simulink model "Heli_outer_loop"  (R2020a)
settings: Solver=FixedStepDiscrete  StartTime=0.0  StopTime=10.0  FixedStep=0.01  RelTol=1e-3  EnableMultiTasking=on
model workspace (MAT data in the model file):
  Ts = 0.01
undefined symbols (not defined in the file or in its folder): DiscIntNeverNeededParam
libraries: simulink x1

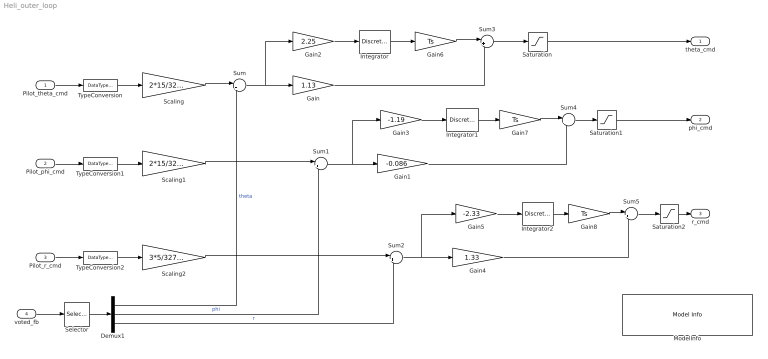
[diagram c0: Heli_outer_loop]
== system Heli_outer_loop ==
  Pilot_theta_cmd : Inport  RequirementInfo={} %GIDa_c6e8f1b9_b611_43b0_b09b_f7299b128b80  OutMin=-32768  OutMax=32767  OutDataTypeStr=int16  PortDimensions=1  SampleTime=0.01
  Pilot_phi_cmd : Inport  RequirementInfo={} %GIDa_de5a2227_6f1d_448c_bc8c_e667ffb26dd8  Port=2  OutMin=-32768  OutMax=32767  OutDataTypeStr=int16  PortDimensions=1  SampleTime=0.01
  Pilot_r_cmd : Inport  RequirementInfo={} %GIDa_bd336e52_072b_4081_8e24_5224b916f056  Port=3  OutMin=-32768  OutMax=32767  OutDataTypeStr=int16  PortDimensions=1  SampleTime=0.01
  voted_fb : Inport  RequirementInfo={} %GIDa_40b9d006_7ccb_49cb_a6ac_aff381845bc4  Port=4  OutMin=-180  OutMax=180  OutDataTypeStr=double  PortDimensions=5  SampleTime=0.01
  Demux1 : Demux  RequirementInfo={} %GIDa_0f7e0ef4_98d4_4326_93b8_613d0164b4b2  Outputs=3
  Gain : Gain  RequirementInfo={} %GIDa_38b33631_7d46_423a_acdb_ff93985993a9  Gain=1.13
  Gain1 : Gain  RequirementInfo={} %GIDa_225d17d5_1a8e_4842_95f8_ce528d38517d  Gain=-0.086
  Gain2 : Gain  RequirementInfo={} %GIDa_ec453ec5_c5c0_44d5_948e_65c93ddaef7c  Gain=2.25
  Gain3 : Gain  RequirementInfo={} %GIDa_943f3cbe_3937_44aa_af38_ec7fec40805c  Gain=-1.19
  Gain4 : Gain  RequirementInfo={} %GIDa_d845b47e_971b_498b_bbe3_d6058df44643  Gain=1.33
  Gain5 : Gain  RequirementInfo={} %GIDa_0a451155_7422_4e41_b41b_ac8de7a0f7bc  Gain=-2.33
  Gain6 : Gain  RequirementInfo={} %GIDa_ec453ec5_c5c0_44d5_948e_65c93ddaef7c  Gain=Ts
  Gain7 : Gain  Gain=Ts
  Gain8 : Gain  Gain=Ts
  Integrator : DiscreteIntegrator  RequirementInfo={} %GIDa_dac8ce2c_b2e5_46af_8a5f_5c149ac95a38  IntegratorMethod=Accumulation: Forward Euler  SampleTime=-1  LimitOutput=on  UpperSaturationLimit=10  LowerSaturationLimit=-10  ICPrevOutput=DiscIntNeverNeededParam  ICPrevScaledInput=DiscIntNeverNeededParam
  Integrator1 : DiscreteIntegrator  RequirementInfo={} %GIDa_c2996118_add0_406e_b8f4_096077f2e691  IntegratorMethod=Accumulation: Forward Euler  SampleTime=-1  LimitOutput=on  UpperSaturationLimit=10  LowerSaturationLimit=-10  ICPrevOutput=DiscIntNeverNeededParam  ICPrevScaledInput=DiscIntNeverNeededParam
  Integrator2 : DiscreteIntegrator  RequirementInfo={} %GIDa_cf0bee46_0c0a_47b2_81ab_c926ffb37de9  IntegratorMethod=Accumulation: Forward Euler  SampleTime=-1  LimitOutput=on  UpperSaturationLimit=10  LowerSaturationLimit=-10  ICPrevOutput=DiscIntNeverNeededParam  ICPrevScaledInput=DiscIntNeverNeededParam
  ModelInfo : simulink/Model-Wide Utilities/Model Info  Frame=on  DisplayStringWithTags=|  HorizontalTextAlignment=Center  LeftAlignmentValue=0.5
      | Model Name: %<ModelName>
      | Model Version: %<ModelVersion>
      | Last Modified: %<LastModificationDate>
      | 
      | Copyright 2016 The MathWorks, Inc.
  Saturation : Saturate  RequirementInfo={} %GIDa_cd349ed3_fa5b_45c3_8aec_effea4668e69  UpperLimit=30  LowerLimit=-30
  Saturation1 : Saturate  RequirementInfo={} %GIDa_cdaf265c_9ec2_4b78_ae7f_0c72f3978ef0  UpperLimit=30  LowerLimit=-30
  Saturation2 : Saturate  RequirementInfo={} %GIDa_b0697b07_104a_4fe5_acf7_d696411481f0  UpperLimit=30  LowerLimit=-30
  Scaling : Gain  Gain=2*15/32767
  Scaling1 : Gain  Gain=2*15/32767
  Scaling2 : Gain  Gain=3*5/32767
  Selector : Selector  RequirementInfo={} %GIDa_e0faeade_0420_4977_bcc4_4057337ee888  InputPortWidth=5  IndexOptions=Index vector (dialog)  Indices=[1 2 3]  OutputSizes=1
  Sum : Sum  RequirementInfo={} %GIDa_aef1367a_fa96_4043_ad47_b91e9938bcbc  Inputs=|+-  InputSameDT=on
  Sum1 : Sum  RequirementInfo={} %GIDa_7cf7cd4c_9daa_4c96_981c_13db01e8d568  Inputs=|+-  InputSameDT=on
  Sum2 : Sum  RequirementInfo={} %GIDa_b75e5239_9c3e_4a2f_9dd4_07e5bc1f13e4  Inputs=|+-  InputSameDT=on
  Sum3 : Sum  RequirementInfo={} %GIDa_dec0004f_1794_4f54_b78d_88f0915d9f6f  Inputs=|++
  Sum4 : Sum  RequirementInfo={} %GIDa_c73371f2_60d8_4f3a_a310_54a28eb8e7bc  Inputs=|++
  Sum5 : Sum  RequirementInfo={} %GIDa_e62dfe4c_4b0b_418d_84f2_d28db5a50898  Inputs=|++
  TypeConversion : DataTypeConversion  OutDataTypeStr=double
  TypeConversion1 : DataTypeConversion  OutDataTypeStr=double
  TypeConversion2 : DataTypeConversion  OutDataTypeStr=double
  theta_cmd : Outport  RequirementInfo={} %GIDa_56ddc0ff_d81c_44a6_a61d_90e8f701c995  VectorParamsAs1DForOutWhenUnconnected=off
  phi_cmd : Outport  RequirementInfo={} %GIDa_10908ca3_1080_4a03_a980_f863f0f9143a  Port=2  VectorParamsAs1DForOutWhenUnconnected=off
  r_cmd : Outport  RequirementInfo={} %GIDa_d0f1d3df_6d10_4b46_9cf8_3e0612fe178e  Port=3  VectorParamsAs1DForOutWhenUnconnected=off
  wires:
  Selector/1 -> Demux1/1
  Demux1/1 -> Sum/2  "theta"
  Demux1/2 -> Sum1/2  "phi"
  Demux1/3 -> Sum2/2  "r"
  voted_fb/1 -> Selector/1
  Sum/1 -> Gain/1, Gain2/1
  Gain/1 -> Sum3/2
  Sum3/1 -> Saturation/1
  Integrator/1 -> Gain6/1
  Gain2/1 -> Integrator/1
  Saturation/1 -> theta_cmd/1
  Sum1/1 -> Gain3/1, Gain1/1
  Gain1/1 -> Sum4/2
  Sum4/1 -> Saturation1/1
  Integrator1/1 -> Gain7/1
  Gain3/1 -> Integrator1/1
  Saturation1/1 -> phi_cmd/1
  Gain4/1 -> Sum5/2
  Sum5/1 -> Saturation2/1
  Integrator2/1 -> Gain8/1
  Gain5/1 -> Integrator2/1
  Sum2/1 -> Gain5/1, Gain4/1
  Saturation2/1 -> r_cmd/1
  TypeConversion2/1 -> Scaling2/1
  TypeConversion1/1 -> Scaling1/1
  TypeConversion/1 -> Scaling/1
  Pilot_theta_cmd/1 -> TypeConversion/1
  Scaling/1 -> Sum/1
  Pilot_phi_cmd/1 -> TypeConversion1/1
  Scaling1/1 -> Sum1/1
  Pilot_r_cmd/1 -> TypeConversion2/1
  Scaling2/1 -> Sum2/1
  Gain6/1 -> Sum3/1
  Gain7/1 -> Sum4/1
  Gain8/1 -> Sum5/1
